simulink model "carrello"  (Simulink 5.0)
settings: Solver=ode45  StartTime=0.0  StopTime=20  RelTol=1e-3
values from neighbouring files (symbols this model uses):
  b = d/2    (= 0.3)    [carrelloParms.m]
  c1 = m0*l*r^3/(4*b^2)    (= 0.136533333333)    [carrelloParms.m]
  c2 = c1    (= 0.136533333333)    [carrelloParms.m]
  kp = 4.154    [carrelloParms.m]
  La = te * Ra    (= 0.0025)    [carrelloParms.m]
  M = [m11, m12; m12 m11]    [carrelloParms.m]
  r = .16    (= 0.16)    [carrelloParms.m]
  Ra = 1    [carrelloParms.m]
  Vs = 50    [carrelloParms.m]

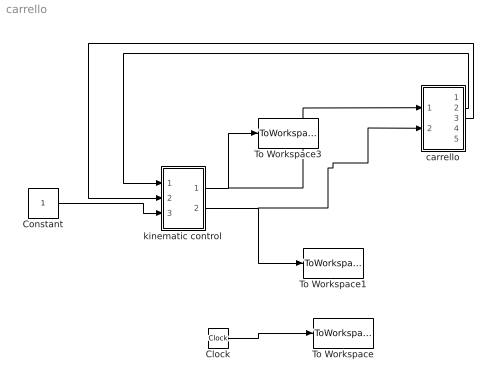
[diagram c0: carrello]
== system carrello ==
  Clock : Clock
  Constant : Constant
  To Workspace : ToWorkspace  VariableName=t  SampleTime=-1  SaveFormat=Array
  To Workspace1 : ToWorkspace  VariableName=vl  SampleTime=-1  SaveFormat=Array
  To Workspace3 : ToWorkspace  VariableName=vr  SampleTime=-1  SaveFormat=Array
  carrello : Subsystem
  kinematic control : Subsystem
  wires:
  Clock/1 -> To Workspace/1
  Constant/1 -> kinematic control/3(vref)
  carrello/3(th) -> kinematic control/2(th)
  carrello/2(y) -> kinematic control/1(y)
  kinematic control/2(Out2) -> carrello/2(vl), To Workspace1/1
  kinematic control/1(Out1) -> carrello/1(vr), To Workspace3/1

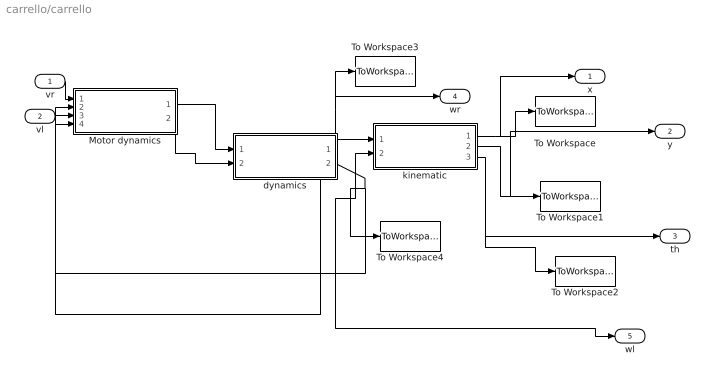
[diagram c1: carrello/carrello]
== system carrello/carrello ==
  vr : Inport
  vl : Inport  Port=2
  Motor dynamics : Subsystem
  To Workspace : ToWorkspace  VariableName=x  SampleTime=-1  SaveFormat=Array
  To Workspace1 : ToWorkspace  VariableName=y  SampleTime=-1  SaveFormat=Array
  To Workspace2 : ToWorkspace  VariableName=th  SampleTime=-1  SaveFormat=Array
  To Workspace3 : ToWorkspace  VariableName=wr  SampleTime=-1  SaveFormat=Array
  To Workspace4 : ToWorkspace  VariableName=wl  SampleTime=-1  SaveFormat=Array
  dynamics : Subsystem
  kinematic : Subsystem
  x : Outport
  y : Outport  Port=2
  th : Outport  Port=3
  wr : Outport  Port=4
  wl : Outport  Port=5
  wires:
  dynamics/1(wr) -> Motor dynamics/3(wr), kinematic/1(wr), To Workspace3/1, wr/1
  dynamics/2(wl) -> Motor dynamics/4(wl), To Workspace4/1, kinematic/2(wl), wl/1
  Motor dynamics/1(tr) -> dynamics/1(tr)
  Motor dynamics/2(tl) -> dynamics/2(tl)
  kinematic/1(x) -> To Workspace/1, x/1
  kinematic/2(y) -> To Workspace1/1, y/1
  kinematic/3(th) -> To Workspace2/1, th/1
  vr/1 -> Motor dynamics/1(vr)
  vl/1 -> Motor dynamics/2(vl)

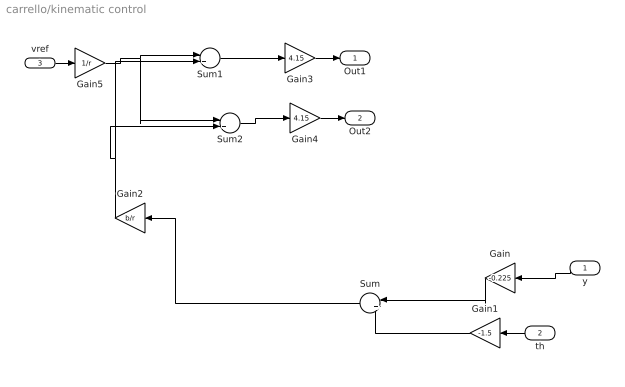
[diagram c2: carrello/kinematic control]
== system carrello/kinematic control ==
  y : Inport  Orientation=left
  th : Inport  Orientation=left  Port=2
  vref : Inport  Port=3
  Gain : Gain  Orientation=left  Gain=-0.225
  Gain1 : Gain  Orientation=left  Gain=-1.5
  Gain2 : Gain  Orientation=left  Gain=b/r
  Gain3 : Gain  Gain=4.15
  Gain4 : Gain  Gain=4.15
  Gain5 : Gain  Gain=1/r
  Sum : Sum  Orientation=left  Inputs=|++
  Sum1 : Sum  Inputs=|++
  Sum2 : Sum  Inputs=|+-
  Out1 : Outport
  Out2 : Outport  Port=2
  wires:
  Gain1/1 -> Sum/2
  Sum/1 -> Gain2/1
  Gain5/1 -> Sum1/1, Sum2/1
  Gain2/1 -> Sum1/2, Sum2/2
  Sum1/1 -> Gain3/1
  Sum2/1 -> Gain4/1
  Gain3/1 -> Out1/1
  Gain4/1 -> Out2/1
  y/1 -> Gain/1
  th/1 -> Gain1/1
  vref/1 -> Gain5/1
  Gain/1 -> Sum/1

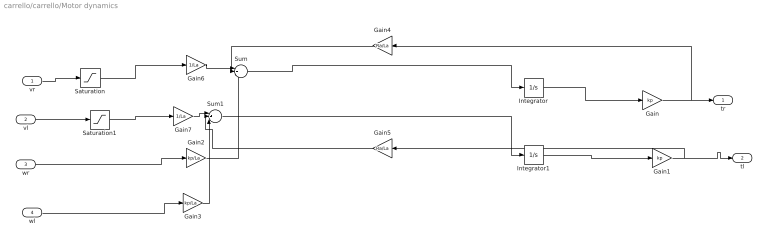
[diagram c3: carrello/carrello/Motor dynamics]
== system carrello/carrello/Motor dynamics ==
  vr : Inport
  vl : Inport  Port=2
  wr : Inport  Port=3
  wl : Inport  Port=4
  Gain : Gain  Gain=kp
  Gain1 : Gain  Gain=kp
  Gain2 : Gain  Gain=kp/La
  Gain3 : Gain  Gain=kp/La
  Gain4 : Gain  Orientation=left  Gain=Ra/La
  Gain5 : Gain  Orientation=left  Gain=Ra/La
  Gain6 : Gain  Gain=1/La
  Gain7 : Gain  Gain=1/La
  Integrator : Integrator
  Integrator1 : Integrator
  Saturation : Saturate  UpperLimit=Vs  LowerLimit=-Vs
  Saturation1 : Saturate  UpperLimit=Vs  LowerLimit=-Vs
  Sum : Sum  Inputs=|+--
  Sum1 : Sum  Inputs=|+--
  tr : Outport
  tl : Outport  Port=2
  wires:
  Gain/1 -> tr/1, Gain4/1
  Gain1/1 -> tl/1, Gain5/1
  Integrator1/1 -> Gain1/1
  Integrator/1 -> Gain/1
  Gain2/1 -> Sum/3
  Sum/1 -> Integrator/1
  wr/1 -> Gain2/1
  wl/1 -> Gain3/1
  Gain3/1 -> Sum1/3
  Gain4/1 -> Sum/2
  Sum1/1 -> Integrator1/1
  Gain5/1 -> Sum1/2
  Gain6/1 -> Sum/1
  Gain7/1 -> Sum1/1
  Saturation/1 -> Gain6/1
  vr/1 -> Saturation/1
  Saturation1/1 -> Gain7/1
  vl/1 -> Saturation1/1

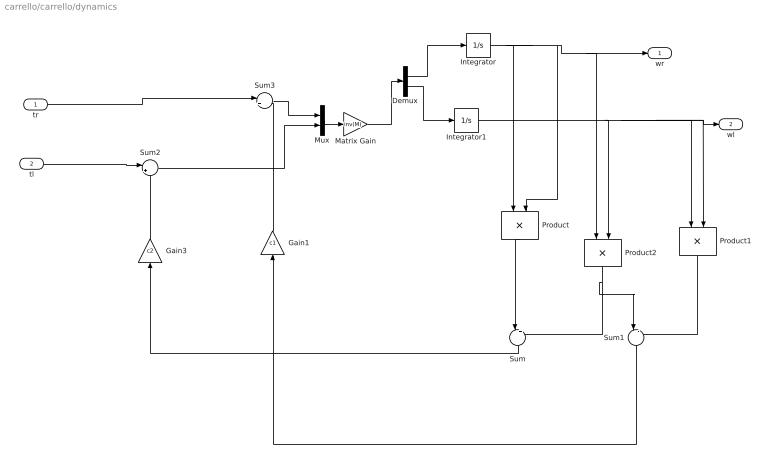
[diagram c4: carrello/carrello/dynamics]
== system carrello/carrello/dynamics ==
  tr : Inport
  tl : Inport  Port=2
  Demux : Demux  Outputs=2
  Gain1 : Gain  Orientation=up  Gain=c1
  Gain3 : Gain  Orientation=up  Gain=c2
  Integrator : Integrator
  Integrator1 : Integrator
  Matrix Gain : Gain  Gain=inv(M)  Multiplication=Matrix(K*u)
  Mux : Mux  Inputs=2
  Product : Product  Orientation=down
  Product1 : Product  Orientation=down
  Product2 : Product  Orientation=down
  Sum : Sum  Orientation=down  Inputs=|+-
  Sum1 : Sum  Orientation=down  Inputs=|-+
  Sum2 : Sum  Inputs=|+-
  Sum3 : Sum  Inputs=|+-
  wr : Outport
  wl : Outport  Port=2
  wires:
  Integrator/1 -> Product/1, Product/2, wr/1, Product2/1
  Integrator1/1 -> Product1/1, wl/1, Product1/2, Product2/2
  Product/1 -> Sum/1
  Product2/1 -> Sum/2, Sum1/1
  Product1/1 -> Sum1/2
  Sum/1 -> Gain3/1
  Sum1/1 -> Gain1/1
  Gain3/1 -> Sum2/2
  tl/1 -> Sum2/1
  Gain1/1 -> Sum3/2
  tr/1 -> Sum3/1
  Sum2/1 -> Mux/2
  Sum3/1 -> Mux/1
  Mux/1 -> Matrix Gain/1
  Matrix Gain/1 -> Demux/1
  Demux/1 -> Integrator/1
  Demux/2 -> Integrator1/1

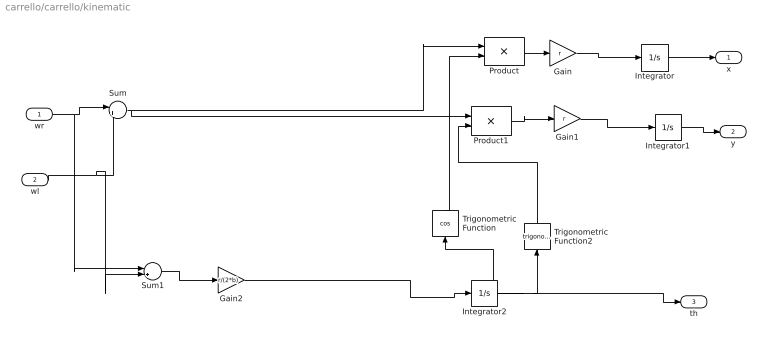
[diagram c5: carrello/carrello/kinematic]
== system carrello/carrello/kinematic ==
  wr : Inport
  wl : Inport  Port=2
  Gain : Gain  Gain=r
  Gain1 : Gain  Gain=r
  Gain2 : Gain  Gain=r/(2*b)
  Integrator : Integrator
  Integrator1 : Integrator
  Integrator2 : Integrator  InitialCondition=pi/4
  Product : Product
  Product1 : Product
  Sum : Sum  Inputs=|++
  Sum1 : Sum  Inputs=|+-
  Trigonometric Function : Trigonometry  Orientation=up  Operator=cos
  Trigonometric Function2 : Trigonometry  Orientation=up
  x : Outport
  y : Outport  Port=2
  th : Outport  Port=3
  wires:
  Integrator/1 -> x/1
  Integrator1/1 -> y/1
  Integrator2/1 -> Trigonometric Function/1, th/1, Trigonometric Function2/1
  Trigonometric Function/1 -> Product/2
  wr/1 -> Sum/1, Sum1/1
  wl/1 -> Sum/2, Sum1/2
  Sum/1 -> Product/1, Product1/1
  Trigonometric Function2/1 -> Product1/2
  Product/1 -> Gain/1
  Product1/1 -> Gain1/1
  Gain1/1 -> Integrator1/1
  Gain/1 -> Integrator/1
  Sum1/1 -> Gain2/1
  Gain2/1 -> Integrator2/1
